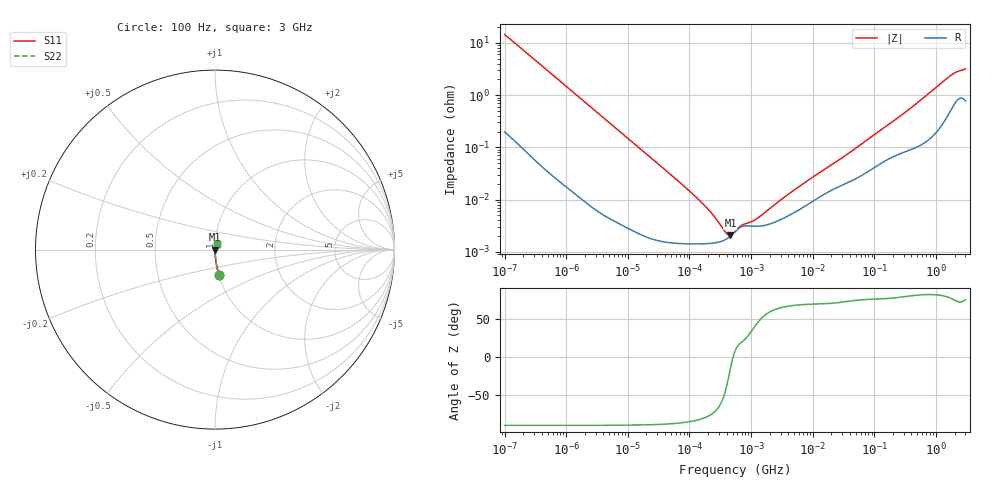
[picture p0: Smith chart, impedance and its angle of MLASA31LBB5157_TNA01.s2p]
! MLASA31LBB5157_TNA01  S-PARAMETER MODEL  ( Standard Model )
! Model Generated by TAIYO YUDEN Corporation (http://www.ty-top.com)
! Version 1.0
! TAIYO YUDEN Control No. 220601
! Copyright(c) 2013 TAIYO YUDEN CO.,LTD. All Rights Reserved.
! Product Description (link to TY-COMPAS)
! https://ds.yuden.co.jp/TYCOMPAS/or/detail?pn=MLASA31LBB5157MTNA01&u=M
! Products Name : Multilayer Ceramic Capacitors
! Characteristics :
!  Capacitance : 150 [uF] , Rated Voltage : 4 [V] , TCC : X5R
!  Case Size : 3.2 x 1.6 / 0.126 x 0.063 [mm/inch] , Thickness : 1.6 / 0.063 [mm/inch]
!  (Conditions: Temperature = 25 [degC] , DC Bias Voltage = 0 [V])
! External Node Assignments :
!  1  o---| |---o  2
! GND o---------o GND
! Frequency Range : 100Hz  -  3GHz  [ 401 STEP ]
# MHZ S RI R 50
! Freq[MHz].  S11 Real  S11 Imag  S21 Real  S21 Imag  S12 Real  S12 Imag  S22 Real  S22 Imag
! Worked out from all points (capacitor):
!   401 points, 100 Hz to 3 GHz, reference 50 ohm
!   read as one part in series: C = 110 uF near 109 Hz
!   lowest |Z| = 2.07 mohm at 461.1 kHz (marker M1)
!   series resonance near 508.5 kHz, so ESL is about 890 pH
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0.0001  0.0223 -0.1411  0.9777 0.1411  0.9777 0.1411  0.0223 -0.1411
0.000114  0.0176 -0.1248  0.9824 0.1248  0.9824 0.1248  0.0176 -0.1248
0.000175  0.00791 -0.0823  0.9921 0.0823  0.9921 0.0823  0.00791 -0.0823
0.000306  0.00284 -0.0475  0.9972 0.0475  0.9972 0.0475  0.00284 -0.0475
0.000664  0.000744 -0.0221  0.9993 0.0221  0.9993 0.0221  0.000744 -0.0221
0.001788  0.000169 -0.00826  0.9998 0.00826  0.9998 0.00826  0.000169 -0.00826
0.031977  1.65e-05 -0.000469  1 0.000469  1 0.000469  1.65e-05 -0.000469
0.126767  1.42e-05 -0.000112  1 0.000112  1 0.000112  1.42e-05 -0.000112
0.138163  1.42e-05 -0.000101  1 0.000101  1 0.000101  1.42e-05 -0.000101
0.157206  1.43e-05 -8.71e-05  1 8.71e-05  1 8.71e-05  1.43e-05 -8.71e-05
0.461094  2e-05 -5.28e-06  1 5.28e-06  1 5.28e-06  2e-05 -5.28e-06
0.547723  2.43e-05 3.53e-06  1 -3.53e-06  1 -3.53e-06  2.43e-05 3.53e-06
2.93481  4.08e-05 8.73e-05  1 -8.73e-05  1 -8.73e-05  4.08e-05 8.73e-05
3.339322  4.39e-05 9.87e-05  1 -9.87e-05  1 -9.87e-05  4.39e-05 9.87e-05
9.794414  9.12e-05 0.000249  0.9999 -0.000249  0.9999 -0.000249  9.12e-05 0.000249
35.62563  0.000208 0.000696  0.9998 -0.000696  0.9998 -0.000696  0.000208 0.000696
175.1444  0.000616 0.00274  0.9994 -0.00274  0.9994 -0.00274  0.000616 0.00274
414.2403  0.000964 0.0059  0.999 -0.0059  0.999 -0.0059  0.000964 0.0059
1714.41  0.00548 0.0228  0.9945 -0.0228  0.9945 -0.0228  0.00548 0.0228
1950.712  0.00707 0.025  0.9929 -0.025  0.9929 -0.025  0.00707 0.025
2219.584  0.00865 0.0266  0.9914 -0.0266  0.9914 -0.0266  0.00865 0.0266
3000  0.00863 0.0302  0.9914 -0.0302  0.9914 -0.0302  0.00863 0.0302
